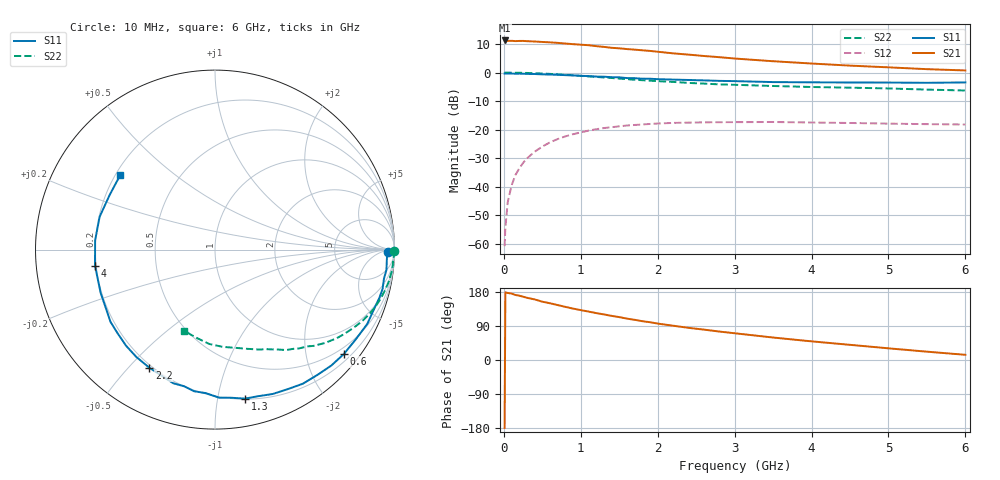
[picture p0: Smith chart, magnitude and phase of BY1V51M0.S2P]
! SIEMENS Small Signal Semiconductors
! BFY420
! Si NPN RF SIEGET Grounded Emitter Transistor in MICRO-X
! VCE = 1.5 V  IC = 1 mA
! Common Emitter S-Parameters:  October  1996
# GHz  S  MA  R  50
!  f  S11  S21  S12  S22
! GHz  MAG  ANG  MAG  ANG  MAG  ANG  MAG  ANG
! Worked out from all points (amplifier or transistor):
!   36 points, 10 MHz to 6 GHz, reference 50 ohm
!   highest |S21| = 11.3 dB at 10 MHz (marker M1)
!   |S21| within 3 dB of that: start of sweep to 1.593 GHz
!   unconditionally stable (mu >= 1): 4.554 GHz to end of sweep
!   at 250 MHz: K = 0.04, MSG = 21.4 dB, |S12| = -31.7 dB
!   at 1.4 GHz: K = 0.21, MSG = 13.9 dB, |S12| = -19.2 dB
!   at 6 GHz: K = 1.34, MAG = 6.0 dB, |S12| = -18.2 dB
!   S11 on the Smith chart (normalised r, x): 10 MHz: 46, -17; 600 MHz: 0.35, -2.78; 1.3 GHz: 0.20, -1.20; 2.2 GHz: 0.19, -0.57; 4 GHz: 0.20, -0.06; 6 GHz: 0.22, +0.33
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0.01  0.9625 -0.8  3.661 -179.4  0.0009 92.5  0.9993 -0.3
0.02  0.9595 -1.6  3.645 178.7  0.0019 95.1  0.9991 -0.7
0.05  0.9591 -3.3  3.593 176.9  0.0053 86.8  0.9976 -1.7
0.1  0.9619 -6.7  3.607 175.3  0.0104 88.6  0.9942 -3.3
0.15  0.9552 -9.8  3.567 171.6  0.0159 83.5  0.9943 -5.1
0.25  0.9545 -16.4  3.596 167.0  0.026 79.0  0.9884 -8.4
0.4  0.9441 -26.0  3.511 159.9  0.0409 74.3  0.9747 -13.3
0.5  0.9301 -32.6  3.445 153.9  0.0503 70.1  0.9626 -16.5
0.6  0.9241 -39.0  3.39 149.7  0.0597 66.5  0.9483 -19.7
0.9  0.8932 -56.8  3.154 135.6  0.083 55.1  0.8952 -28.2
1.1  0.8664 -68.2  3.022 127.8  0.0959 48.5  0.8572 -33.5
1.3  0.8469 -78.6  2.824 120.3  0.1063 42.5  0.8211 -38.1
1.6  0.801 -93.8  2.586 109.2  0.1179 34.5  0.7669 -44.4
1.8  0.7806 -102.7  2.459 102.4  0.123 29.9  0.7349 -47.8
2.2  0.7531 -119.0  2.175 90.5  0.1309 21.6  0.6865 -54.6
2.4  0.7416 -126.2  2.067 84.9  0.1325 18.4  0.6587 -57.7
2.8  0.7153 -139.4  1.864 75.1  0.1347 12.5  0.6211 -63.2
3.5  0.6812 -159.3  1.582 59.3  0.1358 4.8  0.5817 -71.9
4  0.6745 -172.3  1.442 49.2  0.133 0.7  0.5583 -78.5
4.5  0.6699 175.6  1.325 40.0  0.1305 -2.6  0.5438 -85.4
5.5  0.6612 152.6  1.148 22.0  0.1245 -5.9  0.503 -101.5
6  0.6719 141.7  1.09 13.7  0.1227 -5.7  0.4846 -110.7
